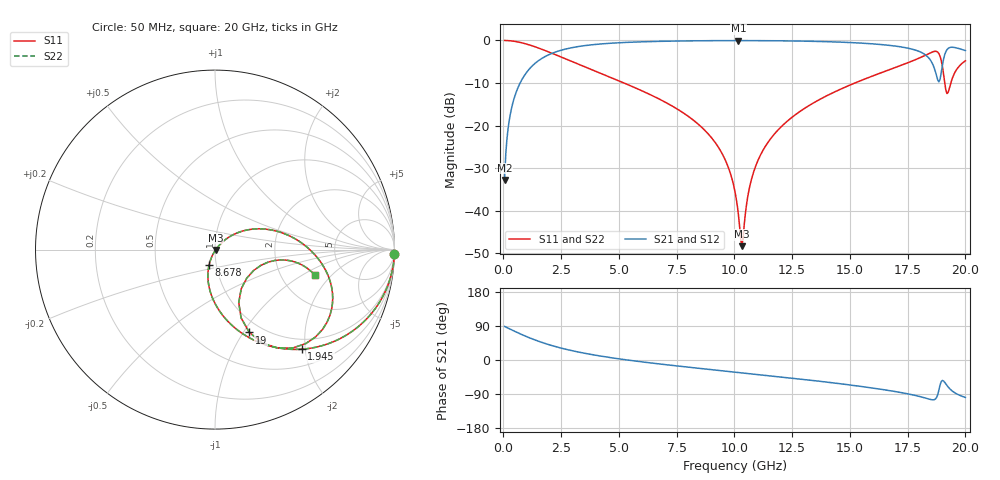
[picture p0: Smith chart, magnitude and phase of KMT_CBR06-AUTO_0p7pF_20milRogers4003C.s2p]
! Data measured by Modelithics Inc. support@modelithics.com 813-866-6335
! KEMET CBR06-AUTO 0.7pF, Pad Width= 0.851mm, Pad Length= 0.64mm, Pad Gap= 0.62mm, 20mil Rogers 4003C substrate Data, January 2022
# hz S ma R 50
! 2 Port Network Data from SP1.SP block
! freq  magS11  angS11  magS21  angS21  magS12  angS12  magS22  angS22
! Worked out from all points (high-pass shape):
!   401 points, 50 MHz to 20 GHz, reference 50 ohm
!   highest |S21| = -0.04 dB at 10.17 GHz (marker M1); lowest = -32.7 dB at 50 MHz (marker M2)
!   |S21| within 3 dB of the highest: 2.097 GHz to 18.17 GHz (16.07 GHz wide, 159 % of centre); 19.13 GHz to end of sweep
!   lowest |S11| = -48.3 dB at 10.32 GHz (marker M3), VSWR 1.01, Z = 50.3 - j0.202 ohm
!   |S11| at or under -10 dB: 5.222 GHz to 15.21 GHz (9.991 GHz wide, 97.8 % of centre); 19.11 GHz to 19.37 GHz (263 MHz wide, 1.37 % of centre)
!   |S22| runs from -48.3 to 0.0 dB; largest |S21 - S12| = 0
!   S11 on the Smith chart (normalised r, x): 50 MHz: 1, -77; 1.945 GHz: 0.80, -1.93; 8.678 GHz: 0.92, -0.16; 19 GHz: 0.87, -1.06; 20 GHz: 3.09, -1.33
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5e7  0.9997 -1.5  0.02307 88.5  0.02307 88.5  0.9997 -1.5
2.99375e8  0.9905 -8.9  0.1369 81.1  0.1369 81.1  0.9905 -8.9
5.98625e8  0.9636 -17.5  0.2668 72.5  0.2668 72.5  0.9636 -17.5
1.94525e9  0.7351 -49.0  0.6765 40.9  0.6765 40.9  0.7351 -49.0
3.391625e9  0.507 -70.6  0.8599 19.2  0.8599 19.2  0.507 -70.6
6.73325e9  0.2057 -99.6  0.9756 -10.3  0.9756 -10.3  0.2057 -99.6
8.678375e9  0.09023 -111.2  0.9924 -23.3  0.9924 -23.3  0.09023 -111.2
9.52625e9  0.04367 -114.1  0.9952 -28.7  0.9952 -28.7  0.04367 -114.1
1.0025e10  0.01669 -109.0  0.9958 -31.9  0.9958 -31.9  0.01669 -109.0
1.017462e10  0.008906 -97.8  0.9958 -32.8  0.9958 -32.8  0.008906 -97.8
1.032425e10  0.003836 -31.5  0.9958 -33.8  0.9958 -33.8  0.003836 -31.5
1.072325e10  0.02258 43.5  0.9954 -36.3  0.9954 -36.3  0.02258 43.5
1.117212e10  0.04759 45.7  0.9943 -39.2  0.9943 -39.2  0.04759 45.7
1.202e10  0.09663 42.5  0.9902 -44.7  0.9902 -44.7  0.09663 42.5
1.336662e10  0.1809 34.3  0.9772 -53.8  0.9772 -53.8  0.1809 34.3
1.670825e10  0.4535 7.4  0.8755 -80.7  0.8755 -80.7  0.4535 7.4
1.785538e10  0.5972 -7.2  0.7673 -93.9  0.7673 -93.9  0.5972 -7.2
1.850375e10  0.7196 -24.6  0.5775 -104.3  0.5775 -104.3  0.7196 -24.6
1.8803e10  0.7279 -46.0  0.3431 -91.3  0.3431 -91.3  0.7279 -46.0
1.90025e10  0.4994 -67.5  0.5068 -54.1  0.5068 -54.1  0.4994 -67.5
1.925188e10  0.245 -28.2  0.8058 -71.1  0.8058 -71.1  0.245 -28.2
2e10  0.5763 -14.5  0.761 -98.8  0.761 -98.8  0.5763 -14.5
